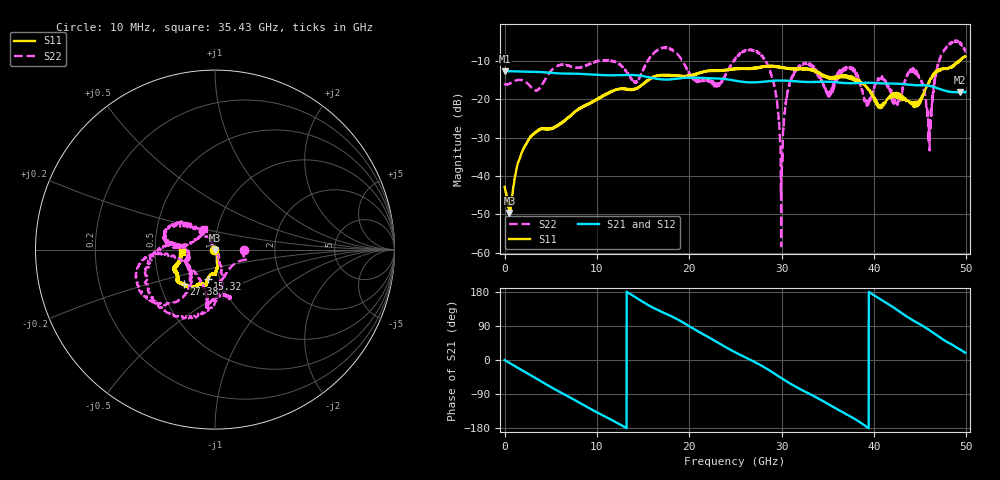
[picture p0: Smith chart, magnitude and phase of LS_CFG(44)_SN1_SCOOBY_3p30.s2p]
!Keysight Technologies,N5245B,MY58422026,A.13.80.08
!Date: Thursday, March 19, 2020 23:40:39
!Correction: S11(Full 2 Port(1,2))
!S21(Full 2 Port(1,2))
!S12(Full 2 Port(1,2))
!S22(Full 2 Port(1,2))
!S2P File: Measurements: S11, S21, S12, S22:
# Hz S DB R 50.0
!freq dBS11 angS11 dBS21 angS21 dBS12 angS12 dBS22 angS22
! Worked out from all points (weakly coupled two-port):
!   4991 points, 10 MHz to 49.91 GHz, reference 50 ohm
!   highest |S21| = -12.59 dB at 20 MHz (marker M1); lowest = -18.1 dB at 49.34 GHz (marker M2)
!   lowest |S11| = -49.7 dB at 530 MHz (marker M3), VSWR 1.01, Z = 49.7 - j0.198 ohm
!   |S11| at or under -10 dB: start of sweep to 49.13 GHz; 49.15674 GHz to 49.23119 GHz (74.45 MHz wide, 0.151 % of centre)
!   |S22| runs from -58.3 to -4.6 dB; largest |S21 - S12| = 0.0022
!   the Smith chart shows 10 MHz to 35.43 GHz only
!   S11 on the Smith chart (normalised r, x): 10 MHz: 0.99, -0.01; 15.32 GHz: 0.87, -0.29; 27.38 GHz: 0.66, -0.27; 35.43 GHz: 0.69, -0.02
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1e7  -42.83 -157.0  -12.59 -0.3  -12.58 -0.3  -15.81 -0.0
2e7  -43.00 -173.2  -12.59 -0.4  -12.58 -0.4  -15.96 -0.5
5.3e8  -49.65 -142.9  -12.62 -7.7  -12.61 -7.6  -15.88 -10.3
2.75e9  -30.02 -54.3  -12.76 -39.0  -12.75 -39.0  -16.42 -25.2
8.33e9  -22.20 -80.8  -13.33 -115.7  -13.32 -115.7  -11.57 -86.5
1.532e10  -15.49 -104.3  -14.04 148.5  -14.02 148.5  -10.75 -175.7
1.665e10  -13.78 -104.8  -14.64 131.3  -14.63 131.3  -6.98 -165.2
2.299e10  -12.52 -117.1  -14.49 47.8  -14.49 47.9  -16.63 -166.4
2.496e10  -12.07 -122.5  -15.05 20.6  -15.04 20.8  -9.59 -175.8
2.738e10  -11.70 -132.0  -15.51 -9.0  -15.50 -8.9  -7.50 -114.8
2.911e10  -11.22 -139.8  -15.10 -34.0  -15.10 -33.9  -15.16 -77.3
2.999e10  -11.76 -142.3  -15.08 -47.8  -15.08 -47.6  -39.93 -4.1
3.103e10  -11.88 -146.4  -15.16 -63.6  -15.17 -63.4  -14.44 135.1
3.328e10  -12.25 -157.9  -15.42 -92.8  -15.42 -92.4  -11.27 172.4
3.543e10  -14.56 -175.5  -15.40 -121.4  -15.35 -120.9  -17.69 118.1
3.723e10  -14.40 173.6  -15.73 -146.0  -15.65 -146.1  -11.89 131.6
4.16e10  -19.39 106.1  -15.84 146.8  -15.86 146.7  -17.05 26.5
4.445e10  -21.16 54.1  -16.28 101.7  -16.29 101.9  -12.36 -19.8
4.602e10  -15.35 6.2  -16.42 78.7  -16.44 78.8  -32.34 -43.2
4.721e10  -12.17 7.8  -17.32 58.8  -17.34 58.9  -8.99 -94.5
4.934e10  -9.85 -16.8  -18.15 27.5  -18.16 27.7  -5.03 -35.9
4.991e10  -8.76 -14.6  -18.06 19.2  -18.08 19.1  -7.40 -23.0
